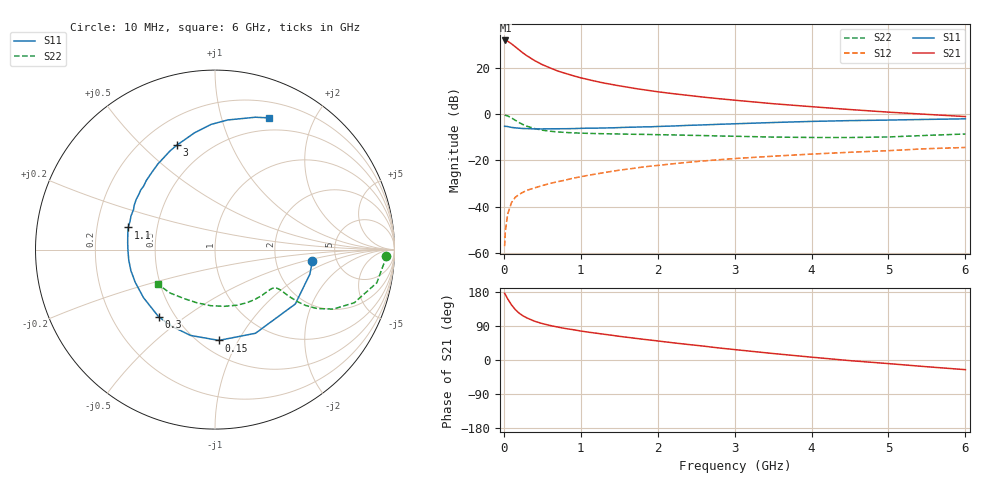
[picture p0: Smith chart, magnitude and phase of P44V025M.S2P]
! SIEMENS Small Signal Semiconductors
! BFP182
! Si NPN RF Bipolar Junction Transistor in SOT143
! VCE = 4 V  IC = 25 mA
! Common Emitter S-Parameters:  March  1996
# GHz  S  MA  R  50
!  f  S11  S21  S12  S22
! GHz  MAG  ANG  MAG  ANG  MAG  ANG  MAG  ANG
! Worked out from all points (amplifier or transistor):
!   36 points, 10 MHz to 6 GHz, reference 50 ohm
!   highest |S21| = 31.9 dB at 20 MHz (marker M1)
!   |S21| within 3 dB of that: start of sweep to 158.5 MHz
!   unconditionally stable (mu >= 1): 674.7 MHz to 5.438 GHz
!   at 250 MHz: K = 0.56, MSG = 30.1 dB, |S12| = -33.8 dB
!   at 1.4 GHz: K = 1.19, MAG = 16.2 dB, |S12| = -24.7 dB
!   at 6 GHz: K = 0.94, MSG = 6.7 dB, |S12| = -14.4 dB
!   S11 on the Smith chart (normalised r, x): 10 MHz: 3.28, -0.61; 150 MHz: 0.61, -0.83; 300 MHz: 0.41, -0.40; 1.1 GHz: 0.34, +0.11; 3 GHz: 0.34, +0.65; 6 GHz: 0.36, +1.43
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0.01  0.5461 -6.8  39.24 176.0  0.0014 82.2  0.9526 -2.0
0.02  0.5461 -14.5  39.28 172.5  0.003 80.2  0.9448 -4.6
0.05  0.5404 -34.1  37.9 161.2  0.0069 79.8  0.9203 -11.6
0.1  0.5179 -64.2  33.18 145.3  0.0123 64.2  0.8303 -20.9
0.15  0.5063 -87.6  28.55 132.8  0.016 58.5  0.7375 -26.7
0.2  0.4974 -106.0  24.45 123.4  0.0185 55.3  0.6572 -30.0
0.25  0.4903 -119.6  20.98 116.4  0.0205 52.7  0.5953 -31.6
0.3  0.4885 -130.1  18.34 111.0  0.0226 51.4  0.5498 -32.2
0.4  0.48 -146.1  14.42 102.3  0.0255 51.7  0.4882 -32.3
0.5  0.4803 -157.7  11.79 96.1  0.0286 52.2  0.4515 -31.9
0.6  0.483 -165.9  10.03 91.2  0.0318 53.4  0.4287 -31.7
0.7  0.484 -173.1  8.595 86.9  0.0347 54.2  0.4133 -31.8
0.8  0.4849 -179.2  7.626 83.1  0.0375 54.9  0.4031 -32.1
1  0.4936 169.9  6.111 76.5  0.0442 55.6  0.3895 -33.3
1.1  0.4992 165.7  5.59 73.4  0.0479 55.8  0.3846 -34.3
1.5  0.5137 151.2  4.105 62.5  0.0615 55.4  0.3729 -39.2
2.2  0.555 129.6  2.777 45.4  0.0847 50.9  0.3561 -51.1
3  0.6197 109.9  2.008 27.5  0.1099 44.0  0.3333 -68.4
3.5  0.6604 100.0  1.685 17.1  0.1234 39.6  0.3201 -80.9
4.5  0.7261 84.3  1.26 -1.7  0.1501 30.7  0.313 -108.7
5.5  0.7712 73.0  0.991 -17.8  0.1794 22.5  0.348 -136.0
6  0.7932 67.7  0.888 -25.5  0.1908 17.5  0.373 -148.9
